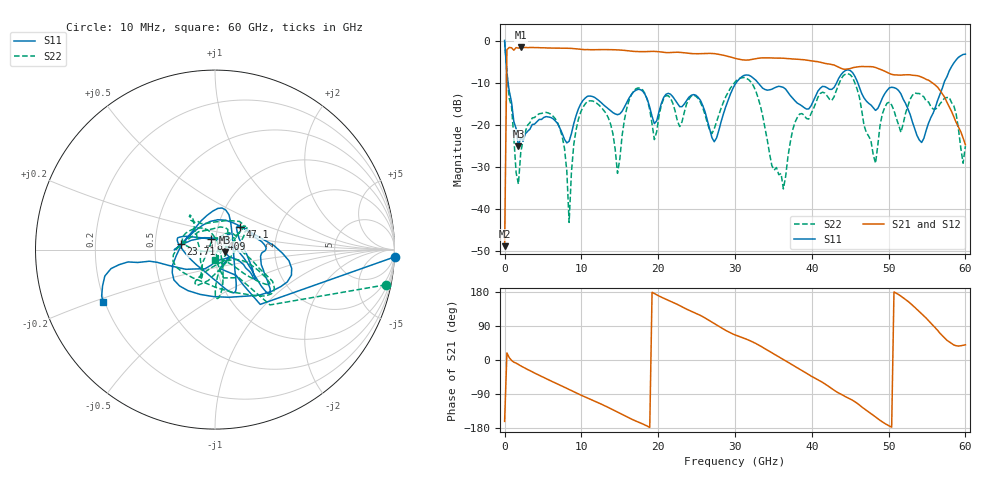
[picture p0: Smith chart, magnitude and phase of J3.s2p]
!Keysight Technologies,N5227A,US51270214,A.10.65.11
!Date: Thursday, October 15, 2020 08:06:47
!Correction: S11(Full 2 Port(1,2))
!S21(Full 2 Port(1,2))
!S12(Full 2 Port(1,2))
!S22(Full 2 Port(1,2))
!S2P File: Measurements: S11, S21, S12, S22:
# Hz S  dB  R 50
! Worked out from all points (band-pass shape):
!   201 points, 10 MHz to 60 GHz, reference 50 ohm
!   highest |S21| = -1.64 dB at 2.11 GHz (marker M1); lowest = -48.9 dB at 10 MHz (marker M2)
!   |S21| within 3 dB of the highest: 294.1 MHz to 31.2 GHz (30.91 GHz wide, 196 % of centre); 31.67 GHz to 39.22 GHz (7.553 GHz wide, 21.3 % of centre)
!   lowest |S11| = -25.2 dB at 1.81 GHz (marker M3), VSWR 1.12, Z = 55.6 - j1.46 ohm
!   |S11| at or under -10 dB: 458.9 MHz to 30.18 GHz (29.72 GHz wide, 194 % of centre); 32.97 GHz to 43.25 GHz (10.28 GHz wide, 27 % of centre); 45.98 GHz to 57.24 GHz (11.26 GHz wide, 21.8 % of centre)
!   |S22| runs from -43.3 to -0.2 dB; largest |S21 - S12| = 0.093
!   S11 on the Smith chart (normalised r, x): 10 MHz: -2, -49; 8.409 GHz: 0.95, +0.11; 23.71 GHz: 0.68, +0.04; 47.1 GHz: 1.28, +0.34; 60 GHz: 0.19, -0.22
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1e7  0.01 -2.3  -48.93 -161.9  -48.60 -163.5  -0.24 -11.6
3.0995e8  -8.05 -50.5  -2.17 18.7  -2.64 25.0  -7.24 -45.1
1.8097e9  -25.18 -13.7  -1.81 -11.9  -1.72 -11.4  -34.16 11.2
2.10965e9  -23.01 7.6  -1.64 -15.4  -1.57 -15.1  -26.66 71.4
6.6089e9  -19.12 46.6  -1.81 -60.5  -1.81 -60.5  -18.62 22.5
7.8087e9  -23.52 68.0  -1.83 -72.0  -1.82 -72.0  -25.69 6.4
8.4086e9  -23.97 109.4  -1.86 -77.9  -1.86 -78.0  -43.27 -70.2
1.02083e10  -14.26 157.8  -2.14 -95.0  -2.14 -95.1  -15.88 172.3
1.470755e10  -17.65 -129.7  -2.22 -137.3  -2.24 -137.3  -31.60 38.9
1.68072e10  -12.19 -71.3  -2.59 -158.5  -2.60 -158.6  -12.02 -83.0
2.010665e10  -16.96 49.1  -2.67 168.9  -2.68 168.9  -17.96 28.3
2.370605e10  -14.29 171.2  -2.99 134.1  -3.00 134.1  -15.07 -102.3
2.730545e10  -24.08 77.1  -3.12 96.2  -3.15 96.2  -20.97 -45.5
3.0005e10  -10.45 -36.4  -4.24 66.2  -4.27 66.2  -9.88 -28.7
3.630395e10  -11.16 5.7  -4.21 1.3  -4.26 1.3  -35.31 -62.4
4.02033e10  -14.37 174.1  -4.88 -45.6  -4.90 -45.8  -16.30 154.1
4.50025e10  -7.13 -13.8  -6.68 -103.1  -6.68 -103.2  -8.14 -32.5
4.710215e10  -14.40 42.4  -6.21 -132.9  -6.23 -132.8  -21.87 39.0
4.830195e10  -16.62 24.9  -6.42 -150.3  -6.47 -150.3  -29.20 173.8
5.010165e10  -11.26 -35.2  -7.84 -174.2  -7.86 -173.9  -14.68 -116.4
5.430095e10  -24.26 -79.5  -8.71 122.4  -8.70 122.3  -13.00 126.9
6e10  -3.25 -154.7  -24.79 40.0  -24.75 40.4  -25.13 -91.8
